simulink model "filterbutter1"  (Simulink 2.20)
settings: Solver=VariableStepDiscrete  StartTime=0.0  StopTime=23  RelTol=1e-3  AbsTol=1e-6
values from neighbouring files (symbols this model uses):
  a = input('Inserisci il dato da graficare [1=PIDNL 2=PD 3=PID]: ')    [grp.m]    (also in grp1.m = input('Inserisci il dato da graficare [1..3]'))
undefined symbols (not defined in the file or in its folder): b, d1, n1

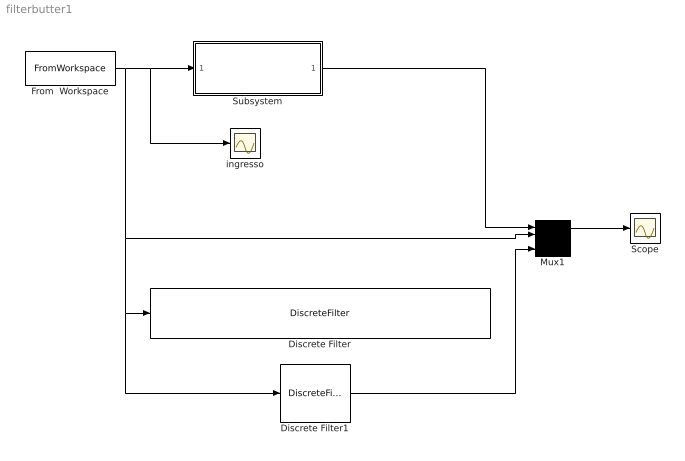
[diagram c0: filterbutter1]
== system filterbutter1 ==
  Discrete Filter : DiscreteFilter  Numerator="[0.0728*10^(-4)    0.2184*10^(-4)   0.2184*10^(-4)     0.0728*10^(-4)  ]"  Denominator="[1.0000   -2.9215    2.8460   -0.9245]"  SampleTime=1
  Discrete Filter1 : DiscreteFilter  Numerator=n1  Denominator=d1  SampleTime=1
  From  Workspace : FromWorkspace  VariableName=[out(:,1),out(:,10)]
  Mux1 : Mux  Inputs=4
  Scope : Scope
  Subsystem : Subsystem  mask(Filtro di Butterworth){ordine=3, freq=0.2/16}
      mask prompts: ordine "Ordine del filtro"; freq "Parametro K per ricavare la Freq. di taglio Ft"
      mask help: Attenzione! Considerare il parametro Fc come la frequanza di campionamento del segnale di ingresso, per cui la frequanza di taglio diviene Ft=K*Fc;
      mask init:
      | [b,a]=butter(ordine,freq);
  ingresso : Scope
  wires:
  From  Workspace/1 -> Mux1/2, Discrete Filter/1, Discrete Filter1/1, Subsystem/1(In1), ingresso/1
  Mux1/1 -> Scope/1
  Discrete Filter1/1 -> Mux1/4
  Subsystem/1(Out1) -> Mux1/1

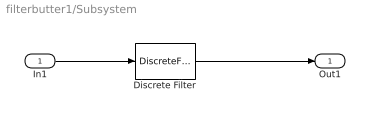
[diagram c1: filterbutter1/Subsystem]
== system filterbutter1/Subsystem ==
  In1 : Inport  Port=1  PortWidth=-1  SampleTime=-1
  Discrete Filter : DiscreteFilter  Numerator=b  Denominator=a  SampleTime=.032
  Out1 : Outport  Port=1
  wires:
  In1/1 -> Discrete Filter/1
  Discrete Filter/1 -> Out1/1
